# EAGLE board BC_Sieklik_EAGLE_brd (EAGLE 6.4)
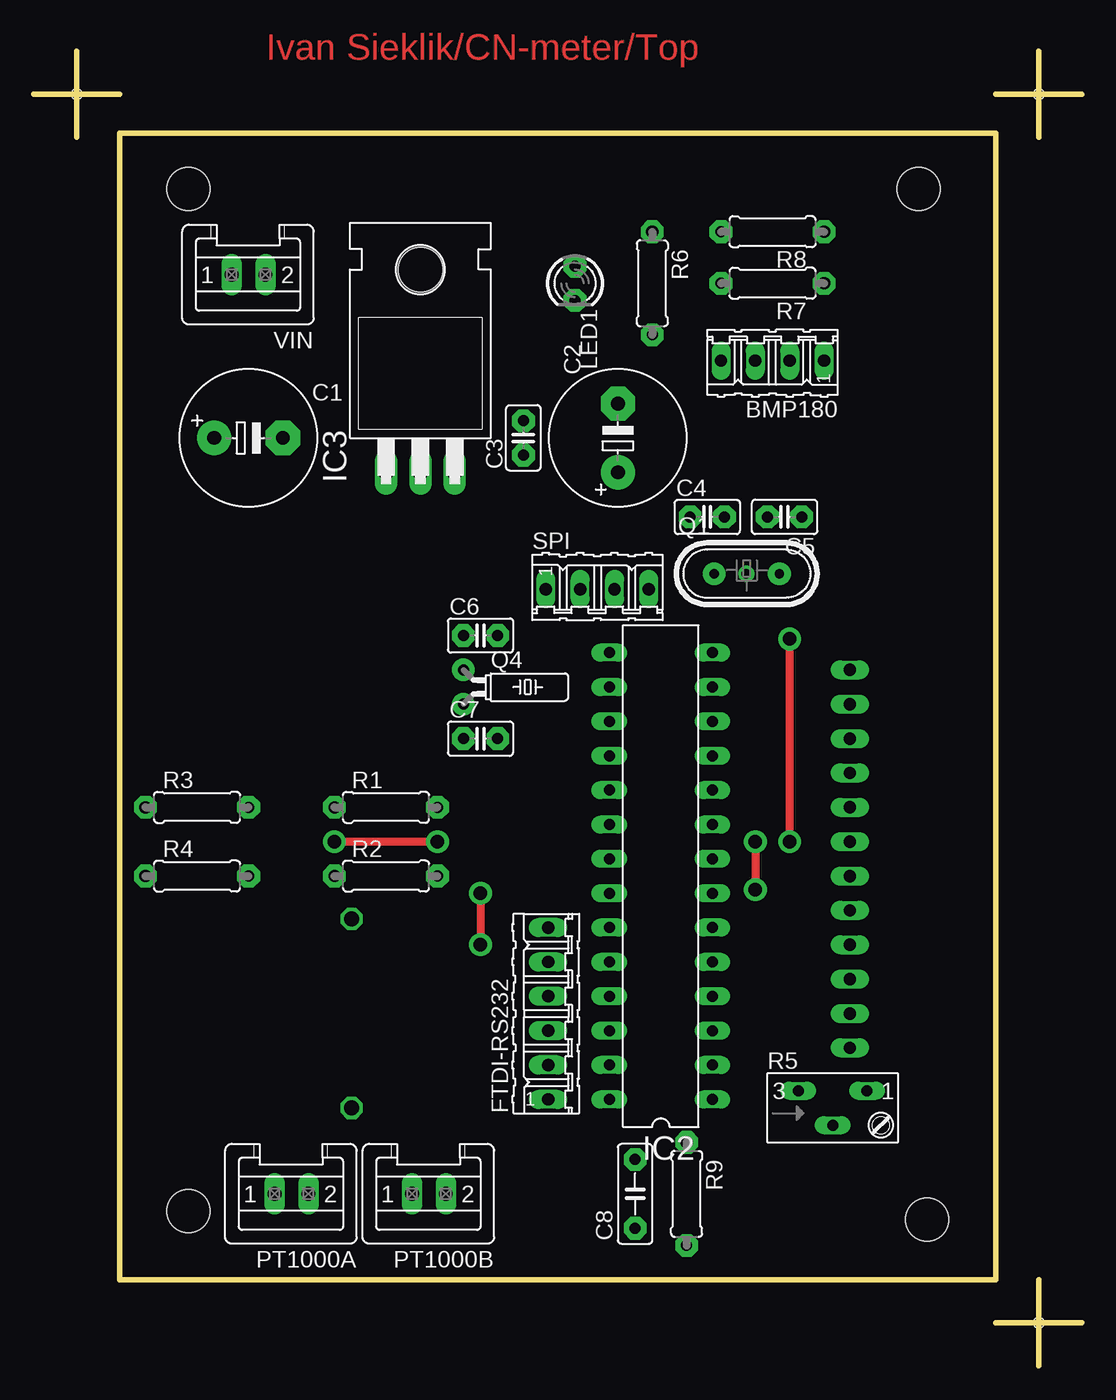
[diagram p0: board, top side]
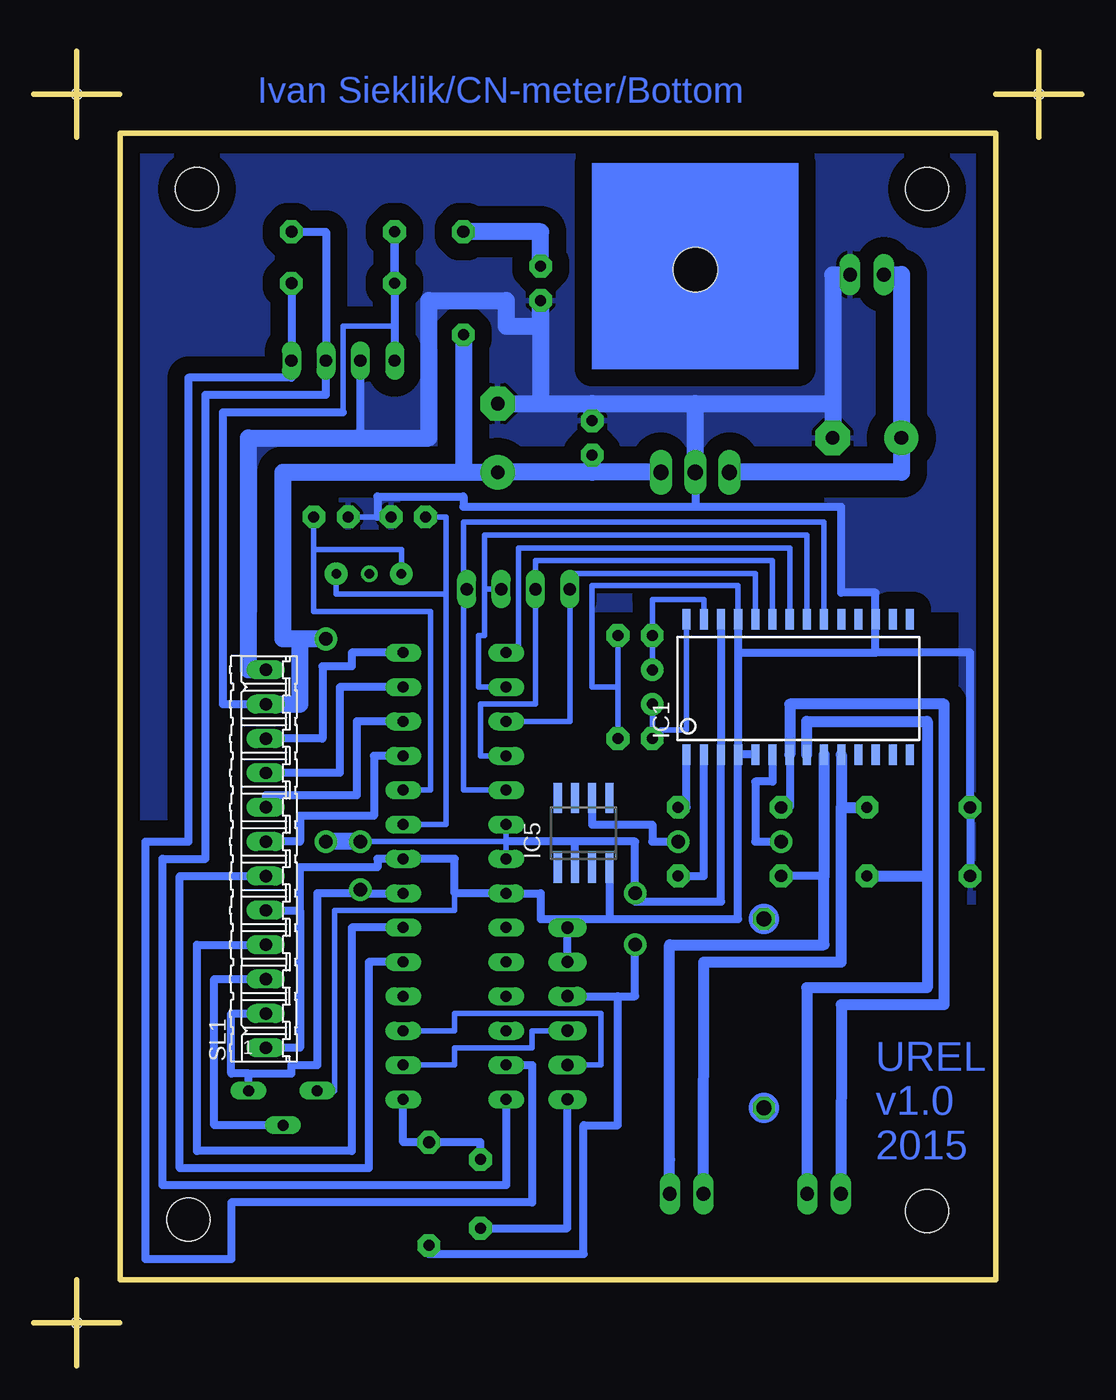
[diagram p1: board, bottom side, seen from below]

Size 77.47 x 97.16 mm. Coordinates in mm from the lower left corner, seen from the top.
Outline: 74.29,97.16 74.29,90.8
Outline: 71.12,93.98 77.47,93.98
Outline: 3.17,97.16 3.17,90.8
Outline: 0,93.98 6.35,93.98
Outline: 74.29,6.35 74.29,0
Outline: 71.12,3.17 77.47,3.17
Outline: 6.35,6.35 71.1,6.35 71.1,91.11 6.35,91.11 6.35,6.35
Copper layers (1*16): Top 0.035mm / dielectric 1.5mm / Bottom 0.035mm
Design rules "default": minimum track width 10mil, minimum drill 24mil, track to track 8mil, track to pad 8mil, pad to pad 8mil, via to via 8mil, smd to smd 8mil, copper to edge 40mil, drill to drill 8mil, minimum pad ring 10mil, minimum via ring 8mil, stop-mask expansion 4mil, vias tented up to drill 0mil, thermal gap 10mil
Holes 3.2 mm at 11.43,86.99 65.41,86.99 66.04,10.79 11.43,11.43
Holes 0.8 mm at 74.29,93.98 3.17,93.98 74.29,3.17
tKeepout: area 6.9,17.5 to 39.9,34.5
tRestrict: area 49.6,73.1 to 59.6,87.1

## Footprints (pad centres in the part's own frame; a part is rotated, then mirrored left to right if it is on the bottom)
04P = drill 0.914 long: 1 -3.81,0; 2 -1.27,0; 3 1.27,0; 4 3.81,0
E5-10,5 = drill 1.016 pad 2.54: + -2.54,0 | drill 1.016 pad 2.54 octagon: - 2.54,0
C025-025X050 = drill 0.813 pad 1.676 octagon: 1 -1.27,0 | drill 0.8 pad 1.676 octagon: 2 1.27,0
C050-025X075 = drill 0.813 pad 1.676 octagon: 1 -2.54,0; 2 2.54,0
06P = drill 0.914 long: 1 -6.35,0; 2 -3.81,0; 3 -1.27,0; 4 1.27,0; 5 3.81,0; 6 6.35,0
SOIC-28 = smd 0.6 x 1.5: 1 -5.715,-5; 2 -4.445,-5; 3 -3.175,-5; 4 -1.905,-5; 5 -0.635,-5; 6 0.635,-5; 7 1.905,-5; 8 3.175,-5; 9 4.445,-5; 10 5.715,-5; 11 6.985,-5; 12 8.255,-5; 13 9.525,-5; 14 10.795,-5; 15 10.795,5; 16 9.525,5; 17 8.255,5; 18 6.985,5; 19 5.715,5; 20 4.445,5; 21 3.175,5; 22 1.905,5; 23 0.635,5; 24 -0.635,5; 25 -1.905,5; 26 -3.175,5; 27 -4.445,5; 28 -5.715,5
DIL28-3 = drill 0.813 long: 1 -16.51,-3.81; 2 -13.97,-3.81; 3 -11.43,-3.81; 4 -8.89,-3.81; 5 -6.35,-3.81; 6 -3.81,-3.81; 7 -1.27,-3.81; 8 1.27,-3.81; 9 3.81,-3.81; 10 6.35,-3.81; 11 8.89,-3.81; 12 11.43,-3.81; 13 13.97,-3.81; 14 16.51,-3.81; 15 16.51,3.81; 16 13.97,3.81; 17 11.43,3.81; 18 8.89,3.81; 19 6.35,3.81; 20 3.81,3.81; 21 1.27,3.81; 22 -1.27,3.81; 23 -3.81,3.81; 24 -6.35,3.81; 25 -8.89,3.81; 26 -11.43,3.81; 27 -13.97,3.81; 28 -16.51,3.81
TO220H = drill 1.118 long: 1 -2.54,-10.16; 2 0,-10.16; 3 2.54,-10.16 | hole 3.302: 0,4.826
SO8 = smd 0.6 x 2.2: 1 -1.905,-2.6; 2 -0.635,-2.6; 3 0.635,-2.6; 4 1.905,-2.6; 5 1.905,2.6; 6 0.635,2.6; 7 -0.635,2.6; 8 -1.905,2.6
LED3MM = drill 0.813 pad 1.676 octagon: A -1.27,0; K 1.27,0
S02P = drill 1.016 long: 1 1.25,0; 2 -1.25,0
HC49U = drill 0.7 pad 1.676: 1 -2.413,0; 3 2.413,0 | drill 0.7 pad 1.2: 2 -0.027,0
TC26H = drill 0.813 pad 1.676: 1 -1.27,0; 2 1.27,0
0207/7 = drill 0.9 pad 1.676 octagon: 1 -3.81,0 | drill 0.813 pad 1.676 octagon: 2 3.81,0
S64Y = drill 0.813 long: A 2.54,1.27; E -2.54,1.27; S 0,-1.27
12P = drill 0.914 long: 1 -13.97,0; 2 -11.43,0; 3 -8.89,0; 4 -6.35,0; 5 -3.81,0; 6 -1.27,0; 7 1.27,0; 8 3.81,0; 9 6.35,0; 10 8.89,0; 11 11.43,0; 12 13.97,0

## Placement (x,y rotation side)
BMP180  [04P]  54.61,74.29 180 top
C1  [E5-10,5]  15.88,68.58 0 top
C2  [E5-10,5]  43.18,68.58 90 top
C3  [C025-025X050]  36.2,68.58 90 top
C4  [C025-025X050]  49.78,62.74 0 top
C5  [C025-025X050]  55.5,62.74 180 top
C6  [C025-025X050]  33.02,53.98 0 top
C7  [C025-025X050]  33.02,46.36 0 top
C8  [C050-025X075]  44.45,12.7 90 top
FTDI-RS232  [06P]  38.02,26.03 90 top
IC1  AD7719  [SOIC-28]  23.49,50.16 0 bottom
IC2  ATmega328P  [DIL28-3]  46.36,36.2 90 top
IC3  7805T  [TO220H]  28.58,76.2 0 top
IC5  AD780R  [SO8]  36.83,39.37 0 bottom
LED1  [LED3MM]  40.01,80.01 270 top
PT1000A  [S02P]  19.05,12.7 180 top
PT1000B  [S02P]  29.21,12.7 180 top
Q1  16MHz  [HC49U]  52.7,58.55 0 top
Q4  [TC26H]  31.75,50.16 270 top
R1  [0207/7]  26.03,41.27 0 top
R2  [0207/7]  26.03,36.2 0 top
R3  [0207/7]  12.06,41.27 0 top
R4  [0207/7]  12.06,36.2 0 top
R5  [S64Y]  59.05,19.05 0 top
R6  [0207/7]  45.72,80.01 270 top
R7  [0207/7]  54.61,80.01 180 top
R8  [0207/7]  54.61,83.82 180 top
R9  [0207/7]  48.26,12.7 270 top
SL1  [12P]  60.33,37.46 90 bottom
SPI  [04P]  41.66,57.4 0 top
VIN  [S02P]  15.88,80.64 180 top

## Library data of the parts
BMP180 FTDI-RS232 SL1 SPI = con-amp-quick; OC_FARNELL: unknown; OC_NEWARK: unknown
C1-C8 R1-R4 R6-R9 = rcl
IC1 = AD7719
IC2 = atmel; OC_FARNELL: unknown; OC_NEWARK: unknown
IC3 = linear
IC5 = analog-devices; MPN: AD780BRZ-REEL; OC_FARNELL: 1464655; OC_NEWARK: 12M8938
LED1 = led; MF: VISHAY SEMICONDUCTOR; OC_FARNELL: 1612437
PT1000A PT1000B VIN = con-amp-mt; OC_FARNELL: unknown; OC_NEWARK: unknown
Q1 Q4 = crystal; OC_FARNELL: unknown; OC_NEWARK: unknown
R5 = pot

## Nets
GND: BMP180.3 C1.- C2.- C3.2 C4.2 C5.2 C6.2 C7.2 FTDI-RS232.5 FTDI-RS232.6 IC1.4 IC1.5 IC1.17 IC1.25 IC2.8 IC2.22 IC3.2 IC5.4 LED1.K R3.1 R4.1 R5.E SL1.1 SL1.5 SL1.12 VIN.2
N$1: C8.1 FTDI-RS232.1
N$2: IC1.2 R2.2
N$3: C7.1 IC1.28 Q4.2
N$4: IC1.8 PT1000A.2 R4.2
N$5: IC1.7 PT1000A.1 R1.1
N$6: IC1.9 PT1000B.2 R2.1
N$7: C8.2 IC2.1 R9.1
N$8: IC1.24 IC2.17 SPI.1
N$9: C5.1 IC2.10 Q1.1
N$10: LED1.A R6.1
N$11: IC1.23 IC2.18 SPI.2
N$12: IC1.20 IC2.19 SPI.4
N$13: IC1.21 IC2.16 SPI.3
N$14: IC1.22 IC2.15
N$15: C6.1 IC1.27 Q4.1
N$16: C1.+ IC3.1 VIN.1
N$17: IC2.14 SL1.10
N$18: FTDI-RS232.3 IC2.2
N$19: C4.1 IC2.9 Q1.3
N$20: IC2.13 SL1.9
N$21: IC2.12 SL1.8
N$22: IC1.10 PT1000B.1 R3.2
N$23: IC2.11 SL1.7
N$24: R5.S SL1.3
N$25: IC2.6 SL1.4
N$26: IC2.5 SL1.6
N$27: BMP180.2 IC2.28 R8.1
N$28: BMP180.1 IC2.27 R7.1
N$29: IC1.1 R1.2
N$30: IC1.6 IC5.6
N$32: FTDI-RS232.2 IC2.3
VCC: BMP180.4 C2.+ C3.1 FTDI-RS232.4 IC1.3 IC1.26 IC2.7 IC2.20 IC2.21 IC3.3 IC5.2 R5.A R6.2 R7.2 R8.2 R9.2 SL1.2 SL1.11

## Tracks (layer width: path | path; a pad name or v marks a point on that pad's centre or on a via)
GND
  Bottom 0.406: IC1.25 25.4,57.66 36.2,57.66 36.2,50.16 34.29,50.16 | C6.2 34.29,50.16 | 34.29,50.16 C7.2 | 46.36,34.92 46.36,33.66 55.25,33.66 55.25,20.32 R5.E | C4.2 52.07,62.74 C5.2
  Bottom 0.61: IC1.25 25.4,52.7 | 25.4,52.7 15.24,52.7 | 25.4,52.7 IC1.4 | 57.79,33.66 57.79,23.49 SL1.1 | 38.1,33.02 40.01,33.02 40.01,34.92 IC2.22 46.36,34.92 46.36,37.46 IC2.8 52.07,37.46 52.07,36.83 57.79,36.83 57.79,33.66 | 38.1,33.02 34.92,33.02 | 34.92,33.02 25.4,33.02 IC1.4 | IC3.2 28.58,63.5 | 28.58,63.5 17.78,63.5 17.78,57.15 15.24,57.15 IC1.17 15.24,52.7 | 15.24,52.7 8.25,52.7 R3.1 R4.1 | 28.58,63.5 45.72,63.5 45.72,64.26 52.07,64.26 52.07,62.74 | BMP180.3 53.34,68.58 | IC5.4 34.92,33.02 | IC1.5 IC1.4 | FTDI-RS232.5 FTDI-RS232.6 38.1,32.38 38.1,33.02 | SL1.5 57.79,33.66
  Bottom 1.27: 18.41,71.12 C1.- | IC3.2 28.58,71.12 | 28.58,71.12 18.41,71.12 | 40.01,71.12 36.2,71.12 | 36.2,71.12 28.58,71.12 | C3.2 36.2,71.12 | 40.01,71.12 LED1.K 40.01,76.83 42.55,76.83 42.55,78.74 48.26,78.74 48.26,68.58 53.34,68.58 61.59,68.58 61.59,51.44 SL1.12 | C2.- 40.01,71.12 | VIN.2 18.41,80.62 18.41,71.12
  pour Bottom (isolate 1.27): 6.35,91.44 6.35,34.29 8.89,34.29 8.89,55.88 66.67,55.88 66.67,39.37 70.48,39.37 70.48,91.44
N$1
  Bottom 0.61: C8.1 38.02,10.16 FTDI-RS232.1
N$2
  Bottom 0.61: R2.2 27.94,36.2 IC1.2
N$3
  Bottom 0.406: IC1.28 29.21,46.99 31.12,46.99 31.12,46.36 C7.1 Q4.2
  Bottom 0.61: IC1.28 29.21,55.25
N$4
  Bottom 0.813: PT1000A.2 20.32,12.7 20.32,27.94 11.43,27.94 11.43,36.2 | IC1.8 20.32,47.62 11.43,47.62 11.43,36.2 | R4.2 11.43,36.2
N$5
  Bottom 0.61: IC1.7 21.59,41.27 R1.1
  Bottom 0.813: PT1000A.1 17.78,26.67 10.16,26.67 10.16,48.9 21.59,48.9 IC1.7
N$6
  Bottom 0.61: 19.05,36.2 R2.1
  Bottom 0.813: IC1.9 19.05,36.2 19.05,31.12 30.48,31.12 30.48,15.24 PT1000B.2
N$7
  Bottom 0.61: IC2.1 50.16,16.51 R9.1 44.45,16.51 C8.2
N$8
  Bottom 0.406: IC1.24 24.13,58.55 37.85,58.55 SPI.1 37.85,47.62 IC2.17
N$9
  Bottom 0.406: 56.77,60.33 56.77,55.75 48.13,55.75 48.13,42.55 IC2.10 | C5.1 56.77,60.33 | 56.77,60.33 50.29,60.33 Q1.1
N$10
  Bottom 1.27: LED1.A 40.01,83.82 R6.1
N$11
  Bottom 0.406: IC1.23 22.86,59.5 40.39,59.5 SPI.2 40.39,48.9 44.45,48.9 44.45,45.09 IC2.18
N$12
  Bottom 0.406: IC1.20 19.05,62.36 45.72,62.36 45.72,57.53 45.72,57.4 | 45.72,57.4 45.72,42.55 IC2.19 | SPI.4 45.72,57.4
N$13
  Bottom 0.406: IC1.21 20.32,61.4 44.13,61.4 44.13,57.4 | 44.13,57.4 44.13,53.98 44.58,53.98 44.58,50.16 IC2.16 | SPI.3 44.13,57.4
N$14
  Bottom 0.406: IC1.22 21.59,60.45 41.66,60.45 41.66,52.7 IC2.15
N$15
  Bottom 0.406: IC1.27 27.94,56.64 31.75,56.64 C6.1 Q4.1
N$16
  Bottom 1.27: VIN.1 13.34,80.66 C1.+ 13.34,66.04 IC3.1
N$17
  Bottom 0.61: SL1.10 56.13,46.36 56.13,51.69 53.98,51.69 53.98,52.7 IC2.14
N$18
  Bottom 0.406: IC2.2 46.36,22.23 46.36,23.49 40.64,23.49 40.64,24.76 FTDI-RS232.3
N$19
  Bottom 0.406: 46.99,57.02 46.99,40.01 IC2.9 | Q1.3 55.12,57.02 46.99,57.02 | C4.1 46.99,62.74 46.99,57.02
N$20
  Bottom 0.61: IC2.13 54.86,50.16 54.86,43.82 SL1.9
N$21
  Bottom 0.61: IC2.12 53.59,47.62 53.59,42.16 60.33,42.16 SL1.8
N$22
  Bottom 0.813: IC1.10 17.78,41.27 | 17.78,41.27 R3.2 | PT1000B.1 27.94,29.84 17.78,29.84 17.78,41.27
N$23
  Bottom 0.61: IC2.11 52.32,45.09 52.32,40.64 57.79,40.64 57.79,38.73 SL1.7
N$24
  Bottom 0.61: R5.S 64.13,17.78 64.13,28.58 SL1.3
N$25
  Bottom 0.61: IC2.6 53.98,32.38 53.98,15.88 65.41,15.88 65.41,31.12 SL1.4
N$26
  Bottom 0.61: IC2.5 52.7,29.84 52.7,14.61 66.67,14.61 66.67,36.2 SL1.6
N$27
  Bottom 0.61: IC2.28 42.55,13.34 67.94,13.34 67.94,37.46 64.77,37.46 64.77,71.75 55.88,71.75 BMP180.2 55.88,83.82 R8.1
N$28
  Bottom 0.61: IC2.27 40.64,22.23 40.64,12.06 62.87,12.06 62.87,7.87 69.22,7.87 69.22,38.73 66.04,38.73 66.04,73.02 58.42,73.02 BMP180.1 R7.1
N$29
  Bottom 0.61: IC1.1 29.21,41.27 R1.2
N$30  (via drill 1 pad 1.68)
  Top 0.61: v22.23,38.73 v29.84,38.73
  Bottom 0.61: IC1.6 22.86,43.18 24.13,43.18 24.13,38.73 v22.23,38.73 | IC5.6 36.2,40.01 31.75,40.01 31.75,38.73 v29.84,38.73
N$31  (via drill 2)
  other vias: 11.43,86.99
N$32
  Bottom 0.406: IC2.3 46.36,24.77 46.36,26.03 35.56,26.03 35.56,22.23 FTDI-RS232.2
N$33  (via drill 1.1)
  other vias: 23.49,33.02
N$34  (via drill 1.1)
  other vias: 23.49,19.05
N$35  (via drill 2)
  other vias: 65.41,86.99
N$36  (via drill 2)
  other vias: 66.04,10.79
N$37  (via drill 2)
  other vias: 11.43,11.43
VCC  (via drill 1 pad 1.68)
  Top 0.61: v55.88,38.73 v55.88,53.72 | v53.34,38.73 v53.34,35.18 | v33.02,34.92 v33.02,31.12
  Bottom 0.406: IC2.21 42.55,38.73 | 42.55,38.73 IC2.20 | 42.55,38.73 v53.34,38.73 | 54.61,70.48 54.61,76.83 50.8,76.83
  Bottom 0.61: IC1.26 IC1.3 26.67,34.29 33.02,34.29 v33.02,34.92 33.02,38.73 37.46,38.73 | 53.34,34.92 56.52,34.92 56.52,22.23 58.42,22.23 58.42,21.59 61.59,21.59 | 61.59,21.59 62.87,21.59 62.87,26.03 SL1.2 | v53.34,35.18 53.34,34.92 | 53.34,34.92 IC2.7 | R5.A 61.59,21.59 | 37.46,38.73 42.55,38.73 | R7.2 R8.2 50.8,76.83 BMP180.4 | 54.61,70.48 63.5,70.48 63.5,48.9 SL1.11 | IC5.2 37.46,38.73 | FTDI-RS232.4 34.29,27.3 | R9.2 48.26,8.25 36.83,8.25 36.83,17.78 34.29,17.78 34.29,27.3 | 34.29,27.3 33.02,27.3 v33.02,31.12
  Bottom 1.27: IC3.3 36.2,66.04 | 36.2,66.04 C2.+ 45.72,66.04 | C3.1 36.2,66.04 | R6.2 45.72,66.04 | 45.72,66.04 59.05,66.04 59.05,53.73 57.79,53.73 | v53.34,38.73 v55.88,38.73 | v55.88,53.72 v55.88,53.73 57.79,53.73 | SL1.11 57.79,48.9 57.79,53.73
(copper drawn outside any net)
  shapes: Bottom area x1, Bottom circle x2

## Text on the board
Top: Ivan Sieklik/CN-meter/Top
Bottom: Ivan Sieklik/CN-meter/Bottom | UREL / v1.0 / 2015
